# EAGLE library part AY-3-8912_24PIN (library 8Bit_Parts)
Dual In Line
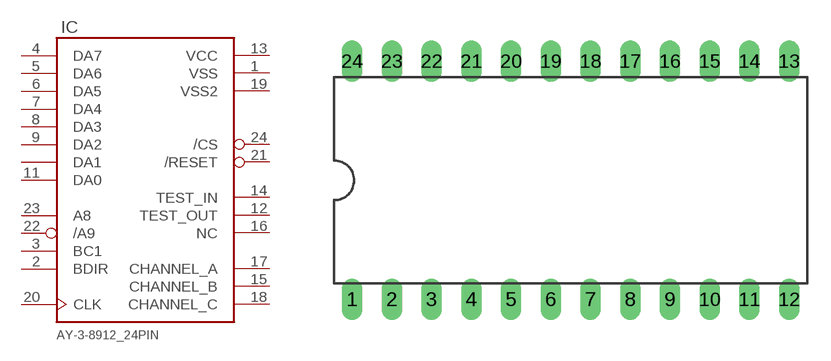
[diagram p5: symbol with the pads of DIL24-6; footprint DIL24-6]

Designator prefix IC

## AY-3-8912_24PIN-6  [DIL24-6]
1  VSS  pwr
2  BDIR  in
3  BC1  in
4  DA7
5  DA6
6  DA5
7  DA4
8  DA3
9  DA2
10  DA1
11  DA0
12  TEST_OUT  nc
13  VCC  pwr
14  TEST_IN  nc
15  CHANNEL_B  out
16  NC  nc
17  CHANNEL_A  out
18  CHANNEL_C  out
19  VSS2  pwr
20  CLK  in
21  /RESET  in
22  /A9  in
23  A8  in
24  /CS  in

## Footprint DIL24-6 (pad centres in mm)
Dual In Line Package 0.6 inch
drill 0.813 long: 1 -13.97,-7.62; 2 -11.43,-7.62; 3 -8.89,-7.62; 4 -6.35,-7.62; 5 -3.81,-7.62; 6 -1.27,-7.62; 7 1.27,-7.62; 8 3.81,-7.62; 9 6.35,-7.62; 10 8.89,-7.62; 11 11.43,-7.62; 12 13.97,-7.62; 13 13.97,7.62; 14 11.43,7.62; 15 8.89,7.62; 16 6.35,7.62; 17 3.81,7.62; 18 1.27,7.62; 19 -1.27,7.62; 20 -3.81,7.62; 21 -6.35,7.62; 22 -8.89,7.62; 23 -11.43,7.62; 24 -13.97,7.62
